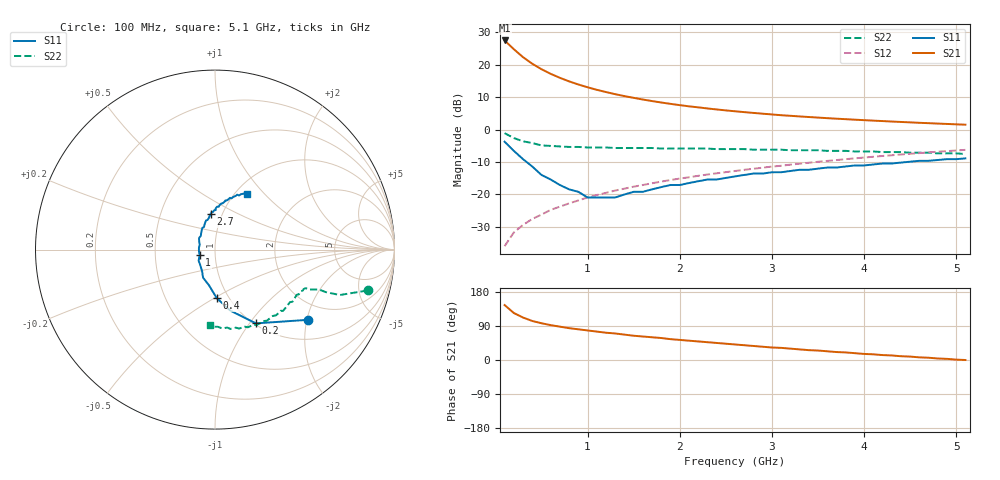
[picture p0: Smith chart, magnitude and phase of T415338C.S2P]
!AT-41533
!S and NOISE PARAMETERS at Vce=8V  Ic=10mA.  LAST UPDATED 01-25-95
# ghz s ma r 50
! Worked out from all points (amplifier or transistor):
!   51 points, 100 MHz to 5.1 GHz, reference 50 ohm
!   highest |S21| = 27.4 dB at 100 MHz (marker M1)
!   |S21| within 3 dB of that: start of sweep to 212.4 MHz
!   unconditionally stable (mu >= 1): 697.1 MHz to 2.19 GHz
!   at 900 MHz: K = 1.03, MAG = 16.9 dB, |S12| = -21.8 dB
!   at 2.6 GHz: K = 0.98, MSG = 9.2 dB, |S12| = -12.8 dB
!   at 5.1 GHz: K = 0.85, MSG = 3.9 dB, |S12| = -6.2 dB
!   lowest NFmin = 0.80 dB at 100 MHz
!   S11 on the Smith chart (normalised r, x): 100 MHz: 1.50, -2.04; 200 MHz: 1.02, -1.07; 400 MHz: 0.88, -0.51; 1 GHz: 0.84, -0.05; 2.7 GHz: 0.88, +0.36; 5.1 GHz: 1.13, +0.81
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0.1  0.65 -37.0  23.58 145.0  0.016 73.0  0.88 -15.0
0.2  0.47 -61.0  17.29 124.0  0.026 68.0  0.74 -20.0
0.3  0.35 -76.0  13.03 112.0  0.034 68.0  0.66 -21.0
0.4  0.27 -88.0  10.32 103.0  0.042 69.0  0.62 -21.0
0.5  0.2 -100.0  8.509 97.0  0.049 69.0  0.57 -23.0
0.6  0.17 -113.0  7.216 92.0  0.058 70.0  0.56 -23.0
0.7  0.14 -121.0  6.266 88.0  0.065 71.0  0.55 -23.0
0.8  0.12 -133.0  5.523 84.0  0.073 71.0  0.54 -24.0
0.9  0.11 -146.0  4.947 81.0  0.081 71.0  0.54 -25.0
1  0.09 -161.0  4.482 78.0  0.09 70.0  0.53 -26.0
1.1  0.09 -173.0  4.095 75.0  0.098 70.0  0.53 -27.0
1.2  0.09 174.0  3.784 72.0  0.106 70.0  0.53 -28.0
1.4  0.1 152.0  3.278 67.0  0.123 69.0  0.52 -30.0
1.6  0.11 136.0  2.903 62.0  0.14 68.0  0.52 -33.0
1.8  0.13 125.0  2.611 58.0  0.158 67.0  0.51 -35.0
2.1  0.15 113.0  2.281 51.0  0.184 65.0  0.51 -39.0
2.6  0.19 99.0  1.914 41.0  0.23 61.0  0.5 -46.0
2.7  0.2 97.0  1.857 39.0  0.24 60.0  0.5 -47.0
3  0.22 91.0  1.71 33.0  0.269 57.0  0.49 -52.0
3.5  0.25 84.0  1.53 25.0  0.319 52.0  0.48 -61.0
4.3  0.3 72.0  1.33 12.0  0.402 44.0  0.45 -77.0
5.1  0.36 60.0  1.189 0.0  0.487 34.0  0.42 -94.0
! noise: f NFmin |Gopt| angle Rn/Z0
0.1  0.8  0.4  8  0.18
0.9  1.1  0.2  93  0.12
1.8  1.5  0.32  -154  0.09
2.4  1.7  0.49  -121  0.17
